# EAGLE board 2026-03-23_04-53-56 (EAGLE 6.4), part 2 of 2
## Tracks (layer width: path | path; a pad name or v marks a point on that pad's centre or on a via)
0  (via drill 0.2 pad 0.48, 0.25 pad 0.56, 0.3 pad 0.66, 2.49 pad 3.48)
  TOP 0.254: 32.77,79.2 32.77,80.64 | 44.96,79.2 44.96,80.64 45.97,81.66 | 57.15,79.2 57.15,80.21 | 69.34,79.2 69.34,80.64 | 80.95,53.47 81.71,54.23 82.55,54.23 v82.68,54.1 | 103.1,76.2 U1.17 103.1,73.41 104.65,71.88 | 102.36,76.96 103.1,76.2 | U1.20 104.6,74.7 104.09,75.21 | 103.1,76.2 104.09,75.21 | 104.09,75.21 105.36,75.21 | 75.04,80.06 75.04,80.9 | 49.89,80.48 50.93,80.48 | 38.21,80.06 38.21,80.9 | 74.79,82.25 74.79,83.08 | 49.76,82.66 50.8,82.66 | 76.96,82.28 78.44,82.28 | 37.44,82.66 38.48,82.66 | 61.95,82.54 62.99,82.54 | 39.62,82.28 41.1,82.28 | 51.82,82.28 53.29,82.28 | 101.33,69.55 101.33,70.38 | 102.72,69.96 103.76,69.96 | 84.18,104.55 84.18,108.58 | 100.46,76.95 104.24,76.95
  TOP 0.508: 38.23,80.49 38.46,80.49 40.39,82.42 | 50.42,80.49 50.77,80.49 52.58,82.3 | 52.58,82.3 54.36,80.52 57.02,80.52 59.05,82.55 62.48,82.55 64.49,82.55 64.77,82.3 | 68.58,41.78 62.61,47.75 36.45,47.75 35.43,48.77 35.43,52.58 36.32,53.47 80.95,53.47 | 62.61,80.49 62.97,80.49 64.77,82.3 | v68.58,31.24 68.58,41.78 | 68.58,41.78 84.58,41.78 | 64.77,82.3 66.55,80.52 69.22,80.52 69.34,80.64 71.37,82.68 74.8,82.68 77.44,82.68 77.72,82.42 | 40.39,82.42 40.11,82.68 37.97,82.68 36.93,81.66 33.78,81.66 32.77,80.64 32.61,80.49 29.08,80.49 27.56,82.02 v27.56,91.82 27.56,101.6 29.08,103.12 84.18,103.12 | 40.39,82.42 40.72,82.75 44.88,82.75 | 45.97,81.66 46.99,82.68 50.29,82.68 52.17,82.68 52.58,82.3 | v99.57,68.83 | v99.57,68.83 99.57,69.98 101.35,69.98 | v101.35,68.83 | v101.35,68.83 101.35,69.98 | 101.35,69.98 103.25,69.98 104.27,69.98 104.65,70.36 104.65,71.88 | 75.06,80.49 75.79,80.49 77.72,82.42 | 81.28,81.41 81.79,80.9 81.79,75.31 84.58,72.52 84.58,41.78 | 81.28,81.41 80.26,82.42 77.72,82.42 | 84.18,103.12 84.2,103.12 91.95,103.12 92.84,104.01 v92.84,109.22 | 84.18,103.12 84.18,106.55 | 81.28,81.41 90.3,90.42 106.3,90.42 107.31,91.44 107.31,95.25 109.22,97.16 114.94,97.16 118.11,100.33 v118.11,109.22 | v101.35,68.83 101.35,45.09 98.04,41.78 84.58,41.78
  BOTTOM 0.254: v82.68,54.1 82.93,54.1 83.69,53.34 | 83.69,53.34 83.82,53.21 | 99.54,77.47 99.54,78.74 | 105.28,85.98 105.28,86.74 105.66,87.12 106.43,87.12 106.78,87.48 106.78,88.27 | 83.69,53.34 83.69,53.57 | 65,82.53 65,84.07 | 79.1,82.4 79.1,83.95 | 38.34,80.31 38.34,81.15 | 70.57,83.8 70.57,84.84 | 71.35,77.81 72.39,77.81 | 58.09,84.31 58.93,84.31 | 50.41,80.31 50.41,81.15 | 34.52,77.81 35.56,77.81 | 46.71,77.81 47.75,77.81 | 34,83.72 34,84.76 | 62.2,80.73 63.25,80.73 | 64.11,80.73 65.15,80.73 | 51.92,80.73 52.96,80.73 | 40.37,80.31 40.37,81.15 | 88.62,86.58 89.66,86.58 | 106.77,87.73 106.77,88.77 | 99.53,76.3 99.53,77.34 | 110.98,69.67 110.98,70.51 | 105.27,77.57 105.27,78.61 | 105.27,81.51 105.27,82.55 | 105.27,79.48 105.27,80.52 | 99.11,80.76 99.95,80.76 | 58.9,77.81 59.94,77.81 | 78.97,49.86 78.97,52.3 | 83.39,53.2 84.23,53.2 | 99.54,76.83
  BOTTOM 0.508: 99.54,79.12 99.54,80.77 99.54,82.27 102.36,85.09 | 35.05,77.83 35.05,82.75 | 40.39,80.75 38.61,80.75 38.61,81.41 38.23,81.79 38.23,83.31 | 47.24,77.83 47.24,82.42 | 59.44,77.83 59.44,82.42 | 50.42,80.75 52.45,80.75 | 50.42,80.75 | 62.74,80.75 | 62.74,80.75 62.74,82.93 62.23,83.44 | v68.58,31.24 68.58,41.91 66.55,43.94 36.96,43.94 35.18,45.72 35.18,52.45 36.45,53.72 77.98,53.72 78.99,52.7 78.99,51.08 | 62.74,80.75 64.64,80.75 | 46.2,82.42 43.31,82.42 42.42,83.31 40.77,83.31 38.23,83.31 | 46.2,82.42 47.24,82.42 | 47.24,82.42 | 46.2,82.42 | 47.24,82.42 | 47.24,82.42 49.4,82.42 50.29,83.29 | 34.01,84.25 34.72,83.57 36.32,83.57 36.58,83.31 | 46.2,82.42 46.2,84.33 | 50.42,80.75 50.42,83.16 50.29,83.29 | 36.58,83.31 36.2,82.93 28.07,82.93 28.07,80.75 27.15,80.75 27.15,80.19 26.98,80.01 26.98,73.2 28.83,71.37 75.82,71.37 76.2,71.37 79.12,74.3 79.12,83.31 76.2,83.31 75.06,82.17 71.88,82.17 | 36.58,83.31 38.23,83.31 | 50.29,83.29 52.93,83.29 52.96,83.31 54.48,83.31 55.37,82.42 58.55,82.42 | 59.44,82.42 | 59.44,82.42 61.21,82.42 62.23,83.44 | 58.55,82.42 59.44,82.42 | 58.55,82.42 58.52,82.42 58.52,84.33 | 62.23,83.44 65.02,83.44 66.8,83.44 68.07,82.17 70.61,82.17 | v101.35,68.83 102.49,67.69 104.01,67.69 v105.16,68.83 | v105.16,68.83 105.16,67.41 106.17,66.42 110.49,66.42 111,66.93 111,70.1 112.27,70.1 113.03,70.87 113.03,74.8 111.76,76.07 105.92,76.07 105.28,76.68 105.28,78.08 | v100.56,76.96 100.43,76.83 99.54,76.83 99.54,77.47 | v105.16,68.83 105.16,70.1 | 71.88,77.83 71.88,82.17 | 70.61,82.17 70.59,82.17 70.59,84.33 | 70.61,82.17 71.88,82.17 | 71.88,82.17 | 99.54,77.47 | 99.54,79.12 | 87.12,86.59 89.15,86.59 91.19,86.59 92.71,85.09 102.36,85.09
  BOTTOM 0.508: v104.14,76.96 105.28,78.08 | 105.28,78.08 105.28,78.11 105.28,80.01 105.28,82.04 105.28,83.95 105.28,85.98 103.25,85.98 102.36,85.09 | 106.78,88.27 109.96,91.44 116.46,91.44 118.11,93.09 v118.11,109.22 | 64.62,80.77 64.64,80.8 | 99.54,77.47 99.54,79.12
  other vias: 80.39,71.37 48.9,48.9 61.47,48.9 52.58,48.9 76.58,48.9 74.8,48.9 63.37,48.9 65.15,48.9 50.8,48.9 38.61,48.9 40.39,48.9 72.9,48.9 36.7,48.9 49.1,81.15 36.02,80.52 31.5,81.69 33.76,80.52 32.61,81.69 61.37,81.15 73.94,81.15 62.99,41.27 65.15,41.27 62.99,38.73 62.99,36.07 62.99,33.4 62.99,30.73 44.93,81.69 48.34,81.69 46.08,80.52 43.81,80.52 43.81,81.69 48.34,80.52 57.1,81.69 60.5,81.69 58.24,80.52 55.98,81.69 60.5,80.52 70.41,80.52 69.27,82.85 72.67,80.52 74.9,81.53 75.77,81.53 76.61,80.39 77.55,80.39 102.36,78.74 102.36,77.75 103.15,76.96 101.55,76.96 102.36,76.15 102.36,75.16 27.3,71.25 30.23,73.15 81.79,71.37 27.3,73.66 41.53,71.37 53.47,71.37 31.5,80.52 34.87,80.52 57.15,80.52 47.19,80.52 55.98,80.52 59.36,80.52 65.91,71.37 68.15,80.52 34.87,81.69 37.03,81.15 36.02,81.69 33.76,81.69 46.08,81.69 47.19,81.69 32.61,82.85 33.76,82.85 27.56,83.44 31.5,82.85 34.87,82.85 36.02,82.85 27.56,85.47 27.56,89.53 43.81,82.85 44.93,82.85 46.08,82.85 48.34,82.85 47.19,82.85 58.24,81.69 59.36,81.69 57.1,82.85 58.24,82.85 55.98,82.85 59.36,82.85 69.27,81.69 68.15,81.69 60.5,82.85 68.15,82.85 70.36,41.27 73.03,41.27 111,68.96 71.53,80.52 72.67,81.69 70.41,81.69 71.53,81.69 70.41,82.85 72.67,82.85 71.53,82.85 73.79,112.39 74.68,112.39 75.56,112.39 62.36,112.39 63.25,112.39 64.14,112.39 64.14,111.12 63.25,111.12 62.36,111.12 75.56,111.12 74.68,111.12 73.79,111.12 85.22,111.25 87,112.39 86.11,111.25 86.11,112.39 85.22,112.39 61.47,111.12 61.47,112.39 87,111.25 60.58,112.39 60.58,111.12 67.69,41.27
  pour TOP (rank 6): 63.83,81.33 63.83,83.24 65.66,83.24 65.66,81.33
  pour TOP (rank 6): 28.37,79.88 28.37,81.08 29.77,81.08 29.77,79.88
  pour TOP (rank 6): 80.01,52.37 80.01,54.28 81.84,54.28 81.84,52.37
  pour TOP (rank 6): 96.52,113.03 96.52,102.87 33.02,102.87 33.02,90.81 28.57,90.81 28.57,83.19 81.28,83.19 81.28,91.44 106.05,91.44 106.05,106.68 111.12,106.68 111.12,113.03 125.73,113.03 125.73,26.67 62.23,26.67 62.23,43.18 34.92,43.18 34.92,54.23 80.52,54.23 80.52,53.59 83.19,53.59 83.19,70.48 78.11,70.48 78.11,80.01 27.94,80.01 27.94,76.2 29.21,76.2 29.21,70.48 26.67,70.48 26.67,113.03
  pour BOTTOM (rank 6): 39.83,82.22 39.83,84.12 41.66,84.12 41.66,82.22
  pour BOTTOM (rank 6): 52.02,82.22 52.02,84.12 53.85,84.12 53.85,82.22
  pour BOTTOM (rank 6): 45.59,83.62 45.59,85.01 46.79,85.01 46.79,83.62
  pour BOTTOM (rank 6): 96.52,113.03 96.52,102.23 33.02,102.23 33.02,85.72 31.75,85.72 31.75,83.31 33.53,83.31 33.53,85.09 34.92,85.09 34.92,84.07 43.05,84.07 43.05,83.19 45.72,83.19 45.72,85.09 46.99,85.09 46.99,84.07 55.24,84.07 55.24,83.19 57.78,83.19 57.78,85.09 59.05,85.09 59.05,84.07 67.56,84.07 67.56,83.31 69.85,83.31 69.85,85.09 71.12,85.09 71.12,84.07 81.28,84.07 81.28,92.08 104.14,92.08 104.14,113.03 125.73,113.03 125.73,26.67 62.87,26.67 62.23,26.67 62.23,43.18 34.92,43.18 34.92,53.98 79.38,53.98 82.17,53.98 82.17,52.07 86.36,52.07 86.36,53.34 90.81,53.34 90.81,55.88 86.36,55.88 86.36,57.15 83.19,57.15 83.19,69.85 26.67,69.85 26.67,113.03
  pour INTERNAL2 (rank 6): 96.52,113.03 26.67,113.03 26.67,79.38 80.64,79.38 80.64,82.55 87.63,82.55 87.63,80.64 103.5,80.64 103.5,92.08 80.64,92.08 80.64,83.19 33.02,83.19 33.02,102.87 96.52,102.87
  pour INTERNAL3 (rank 6): 26.67,70.48 83.19,70.48 83.19,53.98 34.92,53.98 34.92,43.18 62.23,43.18 62.23,26.67 125.73,26.67 125.73,113.03 38.1,113.03 26.67,113.03
  pour INTERNAL1 (rank 6): 26.67,113.03 125.73,113.03 125.73,26.67 26.67,26.67
  pour INTERNAL6 (rank 6): 26.67,113.03 125.73,113.03 125.73,26.67 26.67,26.67
  pour INTERNAL4 (rank 6): 96.52,113.03 26.67,113.03 26.67,26.67 125.73,26.67 125.73,55.88 86.36,55.88 86.36,78.74 28.57,78.74 28.57,84.45 33.66,84.45 33.66,102.23 96.52,102.23
  pour INTERNAL5 (rank 6): 26.67,113.03 96.52,113.03 96.52,102.23 33.02,102.23 33.02,85.72 80.01,85.72 80.01,80.01 26.67,80.01
  pour INTERNAL5 (rank 6): 113.67,113.03 125.73,113.03 125.73,26.67 88.9,26.67 88.9,83.19 113.67,83.19
1  (via drill 0.3 pad 0.66, 2.49 pad 3.48)
  TOP 0.254: 74.79,83.74 74.79,84.58 | 49.76,84.16 50.8,84.16 | 76.96,84.57 78.44,84.57 | 37.44,84.16 38.48,84.16 | 61.95,84.04 62.99,84.04 | 39.62,84.57 41.1,84.57 | 51.82,84.57 53.29,84.57 | 84.18,95.63 84.18,99.67
  TOP 0.508: v102.29,93.98 100.33,95.94 100.33,101.73 | 52.58,84.45 51.44,84.45 51.16,84.18 50.29,84.18 50.19,84.1 49.23,84.1 48.46,84.86 48.46,100.28 49.4,101.22 | 64.77,84.45 63.63,84.45 63.22,84.05 62.48,84.05 62.43,84.1 61.29,84.1 60.66,84.73 60.66,100.15 61.72,101.22 | 73.79,101.22 84.58,101.22 | 84.58,101.22 99.82,101.22 100.33,101.73 | 84.58,101.22 84.18,100.81 84.18,97.66 | 73.79,101.22 72.85,100.28 72.85,84.86 73.61,84.1 74.7,84.1 74.8,84.18 76.05,84.18 76.33,84.45 77.72,84.45 | 49.4,101.22 61.72,101.22 | 100.33,101.73 v100.33,109.22 | 49.4,101.22 38.1,101.22 36.27,99.39 36.27,84.61 36.78,84.1 37.87,84.1 37.97,84.18 38.84,84.18 39.12,84.45 40.39,84.45 | 61.72,101.22 73.79,101.22
  INTERNAL2 0.381: v103.38,68.83 103.38,72.14 105.26,74.02 105.26,92.48 103.76,93.98 v102.29,93.98
  BOTTOM 0.254: 65,84.81 65,86.36 | 79.1,84.68 79.1,86.23 | 102.84,70.09 103.89,70.09
  BOTTOM 0.508: v103.38,68.83 | v103.38,68.83 103.38,70.1
  other vias: 72.85,87 61.72,87 60.71,87 73.79,87 48.46,87 49.48,87 37.21,87 36.32,87 100.46,93.09 91.31,93.98 91.31,93.09 93.09,93.98 93.09,93.09 92.2,93.98 92.2,93.09 80.52,93.98 81.43,93.98 82.35,93.98 80.52,93.09 81.43,93.09 82.35,93.09 100.46,93.98 101.37,93.98 101.37,93.09 102.29,93.09
  pour TOP (rank 2): 63.83,83.62 63.83,85.52 65.66,85.52 65.66,83.62
  pour TOP (rank 4): 80.64,83.82 80.64,92.08 105.41,92.08 105.41,113.03 97.16,113.03 97.16,102.23 33.66,102.23 33.66,90.81 34.92,90.81 34.92,86.36 33.66,86.36 33.66,83.82 41.91,83.82 41.91,86.36 41.27,86.36 41.27,90.81 47.62,90.81 47.62,86.36 45.97,86.36 45.97,83.82 53.34,83.82 53.34,90.81 59.69,90.81 59.69,86.36 58.17,86.36 58.17,83.82 66.04,83.82 66.04,90.81 71.75,90.81 71.75,86.36 70.48,86.36 70.48,83.82
  pour BOTTOM (rank 5): 33.66,85.72 35.56,85.72 35.56,84.45 41.91,84.45 41.91,85.72 47.62,85.72 47.62,84.45 53.98,84.45 53.98,85.72 59.69,85.72 59.69,84.45 66.04,84.45 66.04,85.72 71.75,85.72 71.75,84.45 80.64,84.45 80.64,92.71 103.5,92.71 103.5,113.03 97.16,113.03 97.16,101.6 33.66,101.6
  pour INTERNAL2 (rank 5): 97.16,113.03 97.16,102.23 33.66,102.23 33.66,83.82 80.01,83.82 80.01,92.71 125.73,92.71 125.73,113.03
  pour INTERNAL4 (rank 5): 34.29,101.6 97.16,101.6 97.16,113.03 125.73,113.03 125.73,84.45 34.29,84.45
  pour INTERNAL5 (rank 5): 33.66,101.6 97.16,101.6 97.16,113.03 103.5,113.03 103.5,92.71 80.01,92.71 80.01,86.36 33.66,86.36
2  (via drill 0.25 pad 0.66)
  TOP 0.254: v96.52,79.7 96.55,79.7 97.05,79.2 U1.1
  BOTTOM 0.254: v96.52,79.7 96.14,80.06 96.14,80.77 97.99,80.77 | 97.99,80.77 | 95.71,80.76 96.55,80.76 | 97.61,80.76 98.45,80.76
  pour TOP (rank 3): 99.26,79.1 99.26,79.32 99.52,79.32 99.52,79.1
5  (via drill 0.25 pad 0.66)
  TOP 0.254: v107.95,85.22 104.09,81.36 104.09,79.86
  BOTTOM 0.254: 106.78,85.98 107.54,85.22 v107.95,85.22 108.33,85.22 109.09,85.98 108.71,85.98 | 108.71,85.98 | 108.66,85.97 109.5,85.97
  pour TOP (rank 4): 103.96,79.65 103.96,79.91 104.19,79.91 104.19,79.65
  pour BOTTOM: 106.17,85.27 106.17,86.66 107.37,86.66 107.37,85.27
6  (via drill 0.25 pad 0.66)
  TOP 0.254: 104.6,79.86 104.6,80.59 v107.95,83.95
  BOTTOM 0.254: 109.09,83.95 | v107.95,83.95 109.09,83.95 | v107.95,83.95 | 106.78,83.95 v107.95,83.95 | 106.78,83.95 | 109.08,83.41 109.08,84.45
  pour TOP (rank 4): 104.5,79.65 104.5,79.91 104.72,79.91 104.72,79.65
  pour BOTTOM: 106.17,83.24 106.17,84.63 107.37,84.63 107.37,83.24
7  (via drill 0.25 pad 0.66)
  TOP 0.254: v107.95,82.04 107.95,81.28 105.87,79.2 105.26,79.2
  BOTTOM 0.254: v107.95,82.04 | v107.95,82.04 | v107.95,82.04 109.09,82.04 | 106.78,82.04 v107.95,82.04 | 106.78,82.04 | 109.08,81.51 109.08,82.55 | 106.77,81.51 106.77,82.55
  pour TOP (rank 4): 105.05,79.1 105.05,79.32 105.31,79.32 105.31,79.1
9  (via drill 0.25 pad 0.66)
  TOP 0.254: v107.95,80.01 106.63,78.69 105.26,78.69
  BOTTOM 0.254: 106.78,80.01 v107.95,80.01 109.09,80.01 | 106.78,80.01 | 109.09,80.01 | 109.08,79.48 109.08,80.52 | 106.77,79.48 106.77,80.52
  pour TOP (rank 4): 105.05,78.56 105.05,78.79 105.31,78.79 105.31,78.56
10  (via drill 0.25 pad 0.66)
  TOP 0.254: 105.26,78.21 107.19,78.21 107.31,78.11 v107.95,78.11
  BOTTOM 0.254: 109.09,78.11 | v107.95,78.11 109.09,78.11 | v107.95,78.11 | 106.78,78.11 | 106.78,78.11 v107.95,78.11 | 106.77,77.57 106.77,78.61
  pour TOP (rank 4): 105.05,78.08 105.05,78.31 105.31,78.31 105.31,78.08
  pour BOTTOM: 108.48,77.39 108.48,78.79 109.68,78.79 109.68,77.39
22  (via drill 0.25 pad 0.66)
  TOP 0.254: v102.62,72.9 102.59,72.9 U1.16
  BOTTOM 0.254: 102.84,71.59 103.89,71.59 | 104.65,71.91
  BOTTOM 0.508: v102.62,72.9 102.62,72.36 103.38,71.6 105.16,71.6 | 105.16,71.6
  pour TOP (rank 3): 102.49,73.86 102.49,74.12 102.72,74.12 102.72,73.86
  pour BOTTOM: 104.44,70.99 104.44,72.19 105.84,72.19 105.84,70.99
23  (via drill 0.25 pad 0.66, 0.3 pad 0.66)
  TOP 0.254: 103.5,71.48 103.25,71.48 102.49,72.26 102.23,72.26 v101.85,72.64 101.85,73.15 102.11,73.41 102.11,74.04 | 102.72,71.46 103.76,71.46
  INTERNAL5 0.254: 101.85,71.88 v101.85,72.64
  INTERNAL5 0.508: 101.85,71.88 102.62,71.12 116.08,71.12 119.89,74.93 119.89,97.03 v115.06,101.85 v115.06,102.62
  BOTTOM 0.508: 114.68,102.23 v115.06,101.85 v115.06,102.62 114.68,102.23 | 113.36,102.23 114.68,102.23
  pour TOP (rank 3): 101.98,73.86 101.98,74.12 102.21,74.12 102.21,73.86
  pour BOTTOM: 112.7,101.47 112.7,102.97 114,102.97 114,101.47
24  (via drill 0.3 pad 0.66, 2.49 pad 3.48)
  INTERNAL5 0.508: 108.46,103.25 v110.24,103.25 | v30.23,76.33 v42.42,76.33 v54.61,76.33 v66.8,76.33 70.36,76.33 71.88,77.85 82.3,77.85 84.71,80.26 84.71,82.55 87.63,85.47 104.52,85.47 108.46,89.41 108.46,103.25 | 108.46,103.25 v108.46,109.22
  BOTTOM 0.254: 31.61,75.79 31.61,76.83 | 67.77,76.31 68.61,76.31 | 43.38,76.31 44.22,76.31 | 55.99,75.79 55.99,76.83
  BOTTOM 0.508: v30.23,76.33 | v66.8,76.33 | v66.8,76.33 68.2,76.33 | v54.61,76.33 56.01,76.33 | v42.42,76.33 | v42.42,76.33 43.81,76.33 | v30.23,76.33 31.62,76.33 | v54.61,76.33 | 43.81,76.33 | 31.62,76.33
  BOTTOM 0.762: v110.24,103.25 110.64,103.25 111.66,102.23 | v110.24,102.23 111.66,102.23 | v110.24,101.35 110.77,101.35 111.66,102.23
  pour TOP (rank 5): 106.05,113.03 110.49,113.03 110.49,107.06 106.05,107.06
  pour BOTTOM: 111,101.47 111,102.97 112.29,102.97 112.29,101.47
  pour INTERNAL5 (rank 5): 104.14,113.03 104.14,92.08 80.64,92.08 80.64,79.38 26.67,79.38 26.67,74.93 88.27,74.93 88.27,83.82 113.03,83.82 113.03,113.03
30
  TOP 0.254: U1.11 99.57,74.04 99.19,73.66 96.9,73.66 96.01,72.77 96.01,71.88 96.01,70.87 95.89,70.74 95.89,69.95 | 96,71.35 96,72.39 | 95.87,69.52 95.87,70.36
  pour TOP (rank 2): 99.97,73.86 99.97,74.12 100.2,74.12 100.2,73.86
31  (via drill 0.25 pad 0.66)
  TOP 0.254: 96.47,78.99 v96.52,78.99 96.8,78.69 U1.2
  BOTTOM 0.254: 97.99,78.74 97.74,78.99 v96.52,78.99 | 98.04,76.83 98.04,78.74 | 98.04,76.83 | 98.03,76.3 98.03,77.34
  pour TOP (rank 3): 99.26,78.56 99.26,78.79 99.52,78.79 99.52,78.56
  pour BOTTOM: 97.43,78.03 97.43,79.43 98.63,79.43 98.63,78.03
34  (via drill 0.25 pad 0.66)
  TOP 0.254: v32.77,77.98 33.27,78.49 33.27,79.2
  BOTTOM 0.254: 33.11,75.79 33.11,76.83 | 34.52,76.31 35.56,76.31
  BOTTOM 0.508: v32.77,77.98 33.12,77.6 33.12,76.33 35.05,76.33 | 35.05,76.33
35  (via drill 0.25 pad 0.66)
  TOP 0.254: v44.96,77.98 45.47,78.49 45.47,79.2
  BOTTOM 0.254: 46.71,76.31 47.75,76.31 | 44.88,76.31 45.72,76.31
  BOTTOM 0.508: v44.96,77.98 45.31,77.6 45.31,76.33 45.34,76.33 47.24,76.33
36  (via drill 0.25 pad 0.66)
  TOP 0.254: v57.15,77.98 57.66,78.49 57.66,79.2
  BOTTOM 0.254: 57.49,75.79 57.49,76.83 | 58.9,76.31 59.94,76.31
  BOTTOM 0.508: v57.15,77.98 57.51,77.6 57.51,76.33 57.53,76.33 59.44,76.33
37  (via drill 0.25 pad 0.66)
  TOP 0.254: 69.85,79.2 69.85,78.49 v69.34,77.98
  BOTTOM 0.254: 71.35,76.31 72.39,76.31 | 69.27,76.31 70.1,76.31
  BOTTOM 0.508: 71.88,76.33 69.72,76.33 69.7,76.33 69.7,77.6 v69.34,77.98
38  (via drill 0.25 pad 0.66)
  TOP 0.254: 44.45,79.2 44.45,78.36 v44.07,77.98
  BOTTOM 0.254: 40.37,78.82 40.37,79.65 | 42.15,78.82 42.15,79.65
  BOTTOM 0.508: 40.39,79.25 | 42.16,79.25 | 40.39,79.25 42.16,79.25 | 42.16,79.25 43.43,77.98 v44.07,77.98
39  (via drill 0.25 pad 0.66)
  TOP 0.203: 56.64,79.2 56.64,78.36 v56.26,77.98
  TOP 0.254: 42.42,87.63 42.42,86.74 43.18,85.98 43.76,85.98 44.45,85.29 44.45,84.1 | 41.88,87.62 42.93,87.62
  BOTTOM 0.254: 51.92,79.23 52.96,79.23
  BOTTOM 0.508: 52.45,79.25 54.36,79.25 55.63,77.98 v56.26,77.98 | 52.45,79.25
40  (via drill 0.25 pad 0.66)
  TOP 0.254: Cbst3.2 45.47,86.87 45.47,84.1 | 32.26,79.2 32.26,78.36 v31.88,77.98
  BOTTOM 0.254: 29.44,79.23 30.48,79.23
  BOTTOM 0.508: v31.88,77.98 31.5,77.98 30.2,79.25 29.97,79.25 28.07,79.25 | 28.07,79.25
  pour TOP (rank 2): 45.52,87.02 45.52,88.21 46.91,88.21 46.91,87.02
  pour BOTTOM: 27.36,78.64 27.36,79.83 28.75,79.83 28.75,78.64
41  (via drill 0.25 pad 0.66)
  TOP 0.203: 68.83,79.2 68.83,78.36 v68.45,77.98
  BOTTOM 0.254: 64.11,79.23 65.15,79.23 | 66.55,79.2
  BOTTOM 0.508: 66.55,79.2 66.5,79.25 64.64,79.25 | 66.55,79.25 67.82,77.98 v68.45,77.98
  pour BOTTOM: 65.84,78.64 65.84,79.83 67.23,79.83 67.23,78.64
45  (via drill 0.25 pad 0.66, 0.3 pad 0.66, 1.6 pad 2.21)
  TOP 0.254: v98.53,83.95 98.53,81.81 100.1,80.21 100.1,79.86 | v31.37,85.34 31.77,84.91 31.77,84.1 | v43.56,85.34 43.97,84.91 43.97,84.1 | v110.36,94.11 110.36,92.58 104.52,86.74 104.52,83.19 103.1,81.76 103.1,79.86 | v110.36,89.03 105.16,83.82 105.16,83.19 103.61,81.64 103.61,79.86 | v67.94,85.34 68.35,84.91 68.35,84.1 | 56.16,84.1 56.16,84.91 v55.75,85.34
  INTERNAL5 0.508: v83.19,85.34 v67.94,85.34 67.31,84.71 66.29,84.71 65.66,85.34 v55.75,85.34 55.24,84.84 53.92,84.84 53.42,85.34 v43.56,85.34 | 43.56,85.22 43.56,84.45 43.05,83.95 32.13,83.95 31.37,84.71 v31.37,85.34
  BOTTOM 0.254: v98.53,83.95 92.2,83.95 91.03,85.09 89.15,85.09 87.12,85.09 | 69.08,83.8 69.08,84.84 | 56.59,84.31 57.43,84.31 | 32.5,83.72 32.5,84.76 | 88.62,85.08 89.66,85.08
  BOTTOM 0.508: v83.19,85.34 83.41,85.09 87.12,85.09 | 44.7,84.33 43.94,84.33 43.56,84.71 43.56,85.22 | v31.37,85.34 31.37,84.58 31.67,84.25 32.51,84.25 | v67.94,85.34 67.94,84.58 68.2,84.33 69.09,84.33 | 57.02,84.33 56.01,84.33 55.75,84.58 v55.75,85.34
  pour TOP (rank 3): 99.97,79.65 99.97,79.91 100.2,79.91 100.2,79.65
  pour TOP (rank 4): 103,79.65 103,79.91 103.23,79.91 103.23,79.65
  pour TOP (rank 4): 103.48,79.65 103.48,79.91 103.71,79.91 103.71,79.65
  pour BOTTOM: 86.41,84.48 86.41,85.67 87.81,85.67 87.81,84.48
  pour BOTTOM: 44.09,83.62 44.09,85.01 45.29,85.01 45.29,83.62
56  (via drill 0.25 pad 0.66, 0.3 pad 0.66)
  TOP 0.254: v42.42,77.22 43.97,78.77 43.97,79.2 | 29.08,78.99 29.08,77.6 29.46,77.22 v30.23,77.22 31.77,78.77 31.77,79.2 | 97.51,71.88 97.54,71.86 | U1.13 101.09,73.53 v100.08,72.52 | 68.35,79.2 68.35,78.77 67.56,77.98 67.56,77.47 67.31,77.22 v66.8,77.22 | v54.61,77.22 54.99,77.22 55.63,77.85 55.63,78.23 56.16,78.77 56.16,79.2 | 97.26,69.94 98.3,69.94 | 97.5,71.35 97.5,72.39
  TOP 0.508: 97.51,71.88 98.3,71.88 98.68,71.48 99.57,71.48 100.08,71.98 v100.08,72.52 | 97.54,71.86 97.54,71.02 97.79,70.76 97.79,69.95
  INTERNAL2 0.254: 96.65,72.01 38.86,72.01 33.66,77.22 v30.23,77.22 | 96.65,75.56 83.69,75.56 81.15,73.03 50.04,73.03 45.85,77.22 v42.42,77.22 | 96.14,77.98 83.06,77.98 79.38,74.3 60.96,74.3 58.04,77.22 v54.61,77.22 54.61,77.34 | v94.64,79.48 87.15,79.48 86.23,80.39 83.44,80.39 80.26,77.22 v66.8,77.22
  INTERNAL2 0.508: 96.65,69.09 96.65,75.56 96.65,77.47 96.14,77.98 v94.64,79.48 | 96.65,69.09 v100.08,72.52 | 96.65,69.09 96.65,67.06 98.04,65.66 110.87,65.66 112.14,66.93 v112.14,85.98
  BOTTOM 0.254: 94.59,80.77 94.61,80.75 | 38.34,78.82 38.34,79.65 | 50.41,78.82 50.41,79.65 | 62.2,79.23 63.25,79.23 | 110.16,85.97 111,85.97 | 100.04,70.46 100.04,71.5 | 110.58,83.41 110.58,84.45 | 110.58,81.51 110.58,82.55 | 94.21,80.76 95.05,80.76 | 110.58,79.48 110.58,80.52
  BOTTOM 0.508: 100.08,70.99 v100.08,72.52 | v94.64,79.48 | v94.64,79.48 94.64,80.77 | 62.74,79.25 62.74,78.23 63.75,77.22 v66.8,77.22 | 50.42,79.25 50.42,78.23 51.44,77.22 v54.61,77.22 | 110.59,78.11 110.59,80.01 110.59,82.04 110.59,83.95 110.59,85.98 v112.14,85.98 | v112.14,85.98 | 38.61,79.25 38.41,79.05 38.41,78.28 39.5,77.22 v42.42,77.22
  pour TOP (rank 2): 28.37,78.38 28.37,79.58 29.77,79.58 29.77,78.38
  pour TOP (rank 2): 100.99,73.86 100.99,74.12 101.22,74.12 101.22,73.86
  pour BOTTOM: 109.98,77.39 109.98,78.79 111.18,78.79 111.18,77.39
  pour INTERNAL2 (rank 5): 26.67,78.74 26.67,69.22 83.19,69.22 83.19,55.88 125.73,55.88 125.73,92.08 104.14,92.08 104.14,80.01 87,80.01 87,81.92 81.28,81.92 81.28,78.74
62  (via drill 0.25 pad 0.56, 0.3 pad 0.66, 2.49 pad 3.48)
  TOP 0.254: 80.95,55.5 81.71,54.74 82.55,54.74 v82.68,54.86 | 70.46,66.29 73.28,66.29 | 59.68,65.23 59.68,67.36 | 47.48,65.23 47.48,67.36
  TOP 0.508: v41.66,31.24 41.66,37.08 37.59,41.15 31.5,41.15 29.59,43.05 29.59,53.98 31.11,55.5 80.95,55.5 80.95,63.7 78.33,66.29 71.88,66.29 59.69,66.29 47.5,66.29 35.31,66.29
  BOTTOM 0.254: v82.68,54.86 82.93,54.86 83.82,55.75 | 78.97,56.64 78.97,59.08
  BOTTOM 0.508: 75.82,68.33 28.7,68.33 27.94,67.56 27.94,56.64 29.46,55.12 78.11,55.12 78.99,56.01 78.99,57.86
  other vias: 44.7,41.27 39.12,41.27 41.78,41.27 58.29,41.27 47.5,41.27 50.29,41.27 52.96,41.27 55.63,41.27 59.31,30.73 59.31,33.4 59.31,36.07 59.31,38.73 32.89,60.33 34.67,60.33 36.58,60.33 29.67,66.65 27.3,67.26 27.3,68.2 29.67,64.9 29.67,65.74 42.29,64.9 46.99,60.33 45.21,60.33 48.9,60.33 40.64,64.9 42.29,65.79 57.66,60.33 59.44,60.33 71.75,60.33 61.34,60.33 73.66,60.33 52.96,64.9 54.48,64.9 54.48,65.79 64.9,64.9 69.98,60.33 66.67,65 77.09,64.9 36.45,41.27 40.64,65.79 40.64,66.67 42.29,66.67 52.96,65.79 52.96,66.67 54.48,66.67 64.9,65.79 64.9,66.67 77.09,65.79 66.67,66.7 66.67,65.86 77.09,66.67
  pour TOP (rank 4): 80.01,54.66 80.01,56.57 81.84,56.57 81.84,54.66
  pour TOP (rank 4): 61.59,26.67 61.59,42.55 34.29,42.55 34.29,54.61 80.52,54.61 80.52,55.24 82.55,55.24 82.55,69.85 26.67,69.85 26.67,26.67
  pour BOTTOM: 74.4,67.31 74.4,69.34 77.19,69.34 77.19,67.31
  pour BOTTOM: 83.21,55.04 83.21,56.44 84.4,56.44 84.4,55.04
  pour BOTTOM (rank 5): 26.67,69.22 26.67,26.67 61.59,26.67 61.59,42.55 34.29,42.55 34.29,54.61 82.17,54.61 82.17,69.22
  pour INTERNAL2 (rank 5): 26.67,68.58 82.55,68.58 82.55,55.24 125.73,55.24 125.73,26.67 26.67,26.67
  pour INTERNAL3 (rank 5): 26.67,69.85 26.67,26.67 61.59,26.67 61.59,42.55 34.29,42.55 34.29,54.61 82.55,54.61 82.55,69.85
  pour INTERNAL5 (rank 5): 26.67,74.3 88.27,74.3 88.27,26.67 26.67,26.67
65
  TOP 0.254: 97.79,68.45 98.04,68.45 | 95.89,68.45 97.79,68.45 | 97.79,68.45 | 98.04,68.45 | 98.04,68.45 98.17,68.45 | 96.27,68.58 96.32,68.5 | 96.27,68.58 | 98.04,68.45 98.17,68.58 | 97.26,68.44 98.3,68.44 | 95.87,68.02 95.87,68.86
69  (via drill 0.25 pad 0.66, 0.3 pad 0.66)
  TOP 0.254: 29.97,87.63 29.97,86.87 30.73,86.11 31.75,86.11 32.26,85.57 32.26,84.1 | v100.97,72.64 100.97,72.8 101.6,73.43 U1.14 | 105.26,74.7 105.69,74.7 v106.17,75.18 105.64,75.69 105.26,75.69 | 33.27,84.1 33.27,87.12 33.91,87.76 | 33.9,87.33 33.9,88.16 | 29.96,87.2 29.96,88.04 | 101.33,71.04 101.33,71.88
  TOP 0.381: 101.35,71.48 101.35,72.26 v100.97,72.64
  TOP 0.508: v111,72.64 111,73.53 109.73,74.8 106.55,74.8 v106.17,75.18 | v88.52,65.15 88.52,66.42 | v90.55,65.15 90.55,66.42
  BOTTOM 0.254: 107.05,69.67 107.05,70.51 | 108.95,69.67 108.95,70.51 | 117.31,78.08 117.31,79.12 | 29.44,80.73 30.48,80.73 | 42.15,80.31 42.15,81.15 | 110.98,71.17 110.98,72.01
  BOTTOM 0.508: 111,71.6 v111,72.64 | v107.06,68.83 | v107.06,68.83 107.06,70.1 | 111,71.6 | v108.97,68.96 | v66.55,82.04 | 66.55,80.75 v66.55,82.04 | v54.36,82.04 | 54.36,80.75 v54.36,82.04 | v42.16,82.04 | 42.16,80.75 v42.16,82.04 | v29.97,82.04 | 29.97,80.75 v29.97,82.04 | v108.97,68.96 108.97,70.1 | 117.37,78.61 v118.62,78.61
  pour TOP (rank 2): 89.84,65.81 89.84,67.01 91.24,67.01 91.24,65.81
  pour TOP (rank 2): 101.47,73.86 101.47,74.12 101.7,74.12 101.7,73.86
  pour TOP (rank 3): 105.05,74.57 105.05,74.8 105.31,74.8 105.31,74.57
  pour TOP (rank 3): 105.05,75.59 105.05,75.82 105.31,75.82 105.31,75.59
  pour BOTTOM: 65.84,80.14 65.84,81.33 67.23,81.33 67.23,80.14
  pour INTERNAL4 (rank 5): 125.73,83.82 29.21,83.82 29.21,79.38 87,79.38 87,56.52 125.73,56.52
74
  TOP 0.254: 50.41,76.68 50.41,77.72 | 49.89,78.98 50.93,78.98
  TOP 0.762: 50.42,77.22 50.42,78.99 | 50.42,77.22
75
  TOP 0.254: 62.6,76.68 62.6,77.72
  TOP 0.762: 62.61,77.22 62.61,78.99 | 62.61,78.99
76
  TOP 0.254: 38.21,76.68 38.21,77.72 | 38.21,78.56 38.21,79.4
  TOP 0.762: 38.23,77.22 38.23,78.99 | 38.23,77.22
77
  TOP 0.254: 75.04,78.56 75.04,79.4 | 75.04,76.68 75.04,77.72
  TOP 0.635: 75.06,77.22 | 75.06,77.22 75.06,78.99
78
  TOP 0.254: 43.79,89.12 44.83,89.12
  TOP 0.508: 44.32,89.13 46.05,89.13
  pour TOP (rank 2): 45.52,88.52 45.52,89.71 46.91,89.71 46.91,88.52
79
  TOP 0.254: 58.28,88.7 58.28,89.53 | 55.98,89.12 57.02,89.12 | 58.55,89.18
  TOP 0.508: 56.52,89.13 58.29,89.13 | 58.29,89.13 | 58.29,89.18 58.55,89.18 | 56.52,89.18
80
  TOP 0.254: 33.9,88.82 33.9,89.66 | 31.86,88.82 31.86,89.66 | 31.88,89.26
  TOP 0.508: 33.91,89.26 | 31.88,89.26 33.91,89.26
81
  TOP 0.254: 68.69,88.7 68.69,89.53 | 70.48,89.18
  TOP 0.508: 70.48,89.18 70.43,89.13 68.71,89.13 | 68.71,89.18
  pour TOP (rank 2): 69.77,88.52 69.77,89.71 71.17,89.71 71.17,88.52
84
  TOP 0.254: 72.85,79.2 72.85,78.18 71.88,77.22 71.88,74.4 | 76.54,76.68 76.54,77.72 | 70.46,74.4 73.28,74.4
  TOP 0.762: 76.56,77.22 76.56,75.67 75.29,74.4 71.88,74.4
  pour TOP (rank 5): 66.67,70.48 66.67,76.2 70.48,76.2 70.48,79.38 73.03,79.38 73.03,76.2 77.47,76.2 77.47,70.48
85
  TOP 0.254: 60.66,79.2 60.66,78.31 59.69,77.34 59.69,74.4 | 64.1,76.68 64.1,77.72 | 59.68,73.33 59.68,75.46
  TOP 0.762: 64.11,77.22 64.11,75.29 63.25,74.42 59.69,74.42 59.69,74.4
  pour TOP (rank 5): 65.41,76.2 65.41,70.48 53.98,70.48 53.98,76.2 58.42,76.2 58.42,79.38 60.96,79.38 60.96,76.2
86
  TOP 0.254: 48.46,79.2 48.46,78.44 47.5,77.47 47.5,74.4 | 51.91,76.68 51.91,77.72 | 47.48,73.33 47.48,75.46
  TOP 0.762: 51.92,77.22 51.92,75.54 50.77,74.4 47.5,74.4
  pour TOP (rank 5): 41.91,76.2 41.91,70.48 52.7,70.48 52.7,76.2 48.9,76.2 48.9,79.38 45.85,79.38 45.85,76.2
87
  TOP 0.254: 36.27,79.2 36.27,78.44 35.31,77.47 35.31,74.4 | 39.71,76.68 39.71,77.72
  TOP 0.762: 39.73,77.22 39.73,75.41 38.71,74.4 35.31,74.4
  pour TOP (rank 5): 29.84,70.48 29.84,76.2 33.66,76.2 33.66,79.38 36.83,79.38 36.83,76.2 39.37,76.2 40.64,76.2 40.64,70.48
95
  TOP 0.254: 57.66,84.1 57.66,87 58.29,87.63 | 58.28,87.2 58.28,88.04
107  (via drill 0.25 pad 0.66)
  TOP 0.254: v105.82,72.75 105.54,73.03 104.14,73.03 103.61,73.53 103.61,74.04
  BOTTOM 0.254: v105.82,72.75 106.7,72.75 107.06,72.39 107.06,71.6 | 107.05,71.17 107.05,72.01
  pour TOP (rank 3): 103.48,73.86 103.48,74.12 103.71,74.12 103.71,73.86
108  (via drill 0.3 pad 0.66)
  TOP 0.254: v114.68,78.61 112.52,78.61 111.38,77.47 107.31,77.47 107.06,77.7 105.26,77.7
  BOTTOM 0.254: v114.68,78.61 | v114.68,78.61 115.82,78.61 | 115.81,78.08 115.81,79.12
  pour TOP (rank 4): 105.05,77.6 105.05,77.83 105.31,77.83 105.31,77.6
109  (via drill 0.25 pad 0.66)
  TOP 0.254: v99.19,72.77 99.44,73.03 99.82,73.03 100.61,73.81 100.61,74.04
  BOTTOM 0.254: v99.19,72.77 98.55,72.14 98.55,70.99 | 98.54,70.46 98.54,71.5
  pour TOP (rank 2): 100.48,73.86 100.48,74.12 100.71,74.12 100.71,73.86
110  (via drill 0.25 pad 0.66, 0.3 pad 0.66)
  TOP 0.254: v102.23,86.61 100.41,84.78 100.41,80.92 100.61,80.72 100.61,79.86 | 29.97,89.13 v29.97,90.55 | v29.97,90.55 | 42.42,89.13 v42.42,90.55 | v42.42,90.55 | 54.74,89.13 v54.74,90.55 | v54.74,90.55 | v66.93,90.55 | 66.93,89.13 v66.93,90.55 | 41.88,89.12 42.93,89.12 | 29.96,88.7 29.96,89.53 | 54.2,89.12 55.24,89.12 | 66.92,88.7 66.92,89.53
  BOTTOM 0.254: 105.28,88.27 103.89,88.27 v102.23,86.61 93.6,86.61 89.66,90.55 v66.93,90.55 v54.74,90.55 v42.42,90.55 v29.97,90.55 | 105.27,87.73 105.27,88.77
  pour TOP (rank 3): 100.48,79.65 100.48,79.91 100.71,79.91 100.71,79.65
115  (via drill 0.25 pad 0.56)
  TOP 0.254: v89.92,54.86 90.04,54.74 91.06,54.74 92.46,56.13 92.46,71.48 96.16,75.21 99.44,75.21
  BOTTOM 0.254: v89.92,54.86 89.79,54.74 86.23,54.74 85.45,55.5 85.45,55.63 85.32,55.75
  pour TOP (rank 2): 99.26,75.08 99.26,75.31 99.52,75.31 99.52,75.08
  pour BOTTOM: 84.71,55.04 84.71,56.44 85.9,56.44 85.9,55.04
116  (via drill 0.25 pad 0.56)
  TOP 0.254: v89.92,54.1 90.04,54.23 91.26,54.23 92.96,55.91 92.96,71.27 96.39,74.7 U1.10
  BOTTOM 0.254: v89.92,54.1 89.79,54.23 86.23,54.23 85.45,53.44 85.45,53.34 85.32,53.21 | 84.89,53.2 85.72,53.2
  pour TOP (rank 2): 99.26,74.57 99.26,74.8 99.52,74.8 99.52,74.57
118  (via drill 0.25 pad 0.66)
  TOP 0.254: v106.55,73.36 106.5,73.41 104.39,73.41 104.09,73.69 U1.19
  BOTTOM 0.254: v106.55,73.36 108.1,73.36 108.97,72.52 108.97,71.6 | 108.95,71.17 108.95,72.01
  pour TOP (rank 3): 103.96,73.86 103.96,74.12 104.19,74.12 104.19,73.86
123  (via drill 0.25 pad 0.66, 0.3 pad 0.66)
  TOP 0.254: v102.77,82.96 102.77,82.07 102.59,81.89 102.59,79.86 | 31.27,84.1 30.68,84.1 30.35,84.45 v30.35,85.6
  INTERNAL2 0.254: v30.35,85.6 30.99,86.23 30.99,91.19 32.38,92.58 74.57,92.58 75.46,91.69 88.52,91.69 91.19,89.03 91.19,83.69 91.92,82.96 v102.77,82.96
  pour TOP (rank 4): 102.49,79.65 102.49,79.91 102.72,79.91 102.72,79.65
124  (via drill 0.25 pad 0.66, 0.3 pad 0.66)
  TOP 0.254: v102.21,82.4 102.21,81 102.11,80.9 102.11,79.86 | 43.46,84.1 43,84.1 42.55,84.58 v42.55,85.6
  INTERNAL2 0.254: v42.55,85.6 42.55,89.05 45.41,91.95 74.42,91.95 75.18,91.19 88.14,91.19 90.68,88.65 90.68,83.44 91.72,82.4 v102.21,82.4
  INTERNAL5 0.254: 102.08,82.32 102.11,82.3
  pour TOP (rank 4): 101.98,79.65 101.98,79.91 102.21,79.91 102.21,79.65
125  (via drill 0.25 pad 0.66, 0.3 pad 0.66)
  TOP 0.254: 101.6,79.86 101.6,81.03 101.62,81.05 101.62,81.76 101.6,81.79 | 101.65,81.79 v101.65,81.84 | v54.74,85.6 54.74,84.58 55.19,84.1 55.65,84.1
  INTERNAL2 0.254: v54.74,85.6 54.74,88.65 57.4,91.31 74.3,91.31 74.93,90.68 87.88,90.68 90.17,88.39 90.17,83.19 91.52,81.84 v101.65,81.84
  pour TOP (rank 3): 101.47,79.65 101.47,79.91 101.7,79.91 101.7,79.65
126  (via drill 0.25 pad 0.66, 0.3 pad 0.66)
  TOP 0.254: v101.09,81.28 101.09,81.25 101.09,79.86 | v66.93,85.6 66.93,84.58 67.39,84.1 67.84,84.1
  INTERNAL2 0.254: v66.93,85.6 66.93,88.77 68.33,90.17 87.63,90.17 89.66,88.14 89.66,83.06 91.44,81.28 v101.09,81.28
  pour TOP (rank 3): 100.99,79.65 100.99,79.91 101.22,79.91 101.22,79.65
127  (via drill 2.49 pad 3.48)
  TOP 0.254: v123.19,80.64 119.38,76.83 107.01,76.83 106.63,77.19 105.26,77.19
  pour TOP (rank 4): 105.05,77.09 105.05,77.32 105.31,77.32 105.31,77.09
128  (via drill 2.49 pad 3.48)
  TOP 0.254: v123.19,70.48 117.98,75.69 106.68,75.69 106.15,76.2 105.26,76.2
  pour TOP (rank 4): 105.05,76.07 105.05,76.3 105.31,76.3 105.31,76.07
129  (via drill 2.49 pad 3.48)
  TOP 0.254: v123.19,75.56 119.76,75.56 119,76.33 106.81,76.33 106.4,76.71 105.26,76.71
  pour TOP (rank 4): 105.05,76.58 105.05,76.81 105.31,76.81 105.31,76.58
134  (via drill 0.25 pad 0.66, 0.3 pad 0.66)
  TOP 0.254: 99.44,76.71 94.23,76.71 86.74,69.22 v85.72,69.22 | v30.23,77.98 30.23,78.74 30.68,79.2 31.27,79.2
  INTERNAL2 0.254: v30.23,77.98 29.34,77.98 28.7,77.34 28.7,71.17 29.64,70.23 83.31,70.23 84.33,69.22 v85.72,69.22
  pour TOP (rank 3): 99.26,76.58 99.26,76.81 99.52,76.81 99.52,76.58
135  (via drill 0.25 pad 0.66, 0.3 pad 0.66)
  TOP 0.254: U1.5 93.95,77.19 90.93,74.17 v85.72,74.17 | 43.46,79.2 42.75,79.2 42.42,78.87 v42.42,77.98
  INTERNAL2 0.254: v42.42,77.98 41.66,77.98 41.02,77.34 41.02,73.41 41.91,72.52 82.8,72.52 84.45,74.17 v85.72,74.17
  pour TOP (rank 3): 99.26,77.09 99.26,77.32 99.52,77.32 99.52,77.09
136  (via drill 0.25 pad 0.66, 0.3 pad 0.66)
  TOP 0.254: U1.4 93.83,77.7 92.96,76.83 v85.72,76.83 | v54.61,77.98 54.61,78.61 55.19,79.2 55.65,79.2
  INTERNAL2 0.254: v54.61,77.98 53.85,77.98 53.21,77.34 53.21,74.17 53.72,73.66 79.86,73.66 83.03,76.83 v85.72,76.83
  pour TOP (rank 3): 99.26,77.6 99.26,77.83 99.52,77.83 99.52,77.6
137  (via drill 0.25 pad 0.66, 0.3 pad 0.66)
  TOP 0.254: 99.44,78.21 93.34,78.21 92.2,79.38 v85.72,79.38 | 67.84,79.2 67.39,79.2 66.8,78.61 v66.8,77.98
  INTERNAL2 0.254: v66.8,77.98 66.04,77.98 65.41,77.34 65.41,75.69 66.17,74.93 78.99,74.93 83.44,79.38 v85.72,79.38
  pour TOP (rank 3): 99.26,78.08 99.26,78.31 99.52,78.31 99.52,78.08
140
  TOP 0.254: 56.52,87.63 57.15,86.97 57.15,84.1 | 55.98,87.62 57.02,87.62
144
  TOP 0.254: 68.71,87.63 69.34,86.97 69.34,84.1 | 68.69,87.2 68.69,88.04
145
  TOP 0.254: 69.85,84.1 69.85,87 70.48,87.63
  pour TOP (rank 2): 69.77,87.02 69.77,88.21 71.17,88.21 71.17,87.02
146
  TOP 0.254: 66.93,87.63 66.93,86.74 67.56,86.08 68.45,86.08 68.83,85.7 68.83,84.1 | 66.92,87.2 66.92,88.04
148
  TOP 0.254: 54.74,87.63 54.74,86.61 55.42,85.93 56.06,85.93 56.64,85.32 56.64,84.1 | 54.2,87.62 55.24,87.62
150
  TOP 0.254: 32.77,84.1 32.77,86.84 31.88,87.76 | 31.86,87.33 31.86,88.16
155
  TOP 0.254: 44.96,84.1 44.96,86.97 44.32,87.63 | 43.79,87.62 44.83,87.62
158
  TOP 0.254: 88.52,67.92 88.52,70.23 94.49,76.2 U1.7
  pour TOP (rank 2): 99.26,76.07 99.26,76.3 99.52,76.3 99.52,76.07
159
  TOP 0.254: U1.8 94.61,75.69 90.55,71.63 90.55,67.92
  pour TOP (rank 2): 89.84,67.31 89.84,68.5 91.24,68.5 91.24,67.31
  pour TOP (rank 2): 99.26,75.59 99.26,75.82 99.52,75.82 99.52,75.59

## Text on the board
ASSYNOTES: Cin | Coutx_ch1 | Design Rules: | Min Clearance: 10mil | Min Track Width: 10mil
bDocu: Coutx_ch2 | Cout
